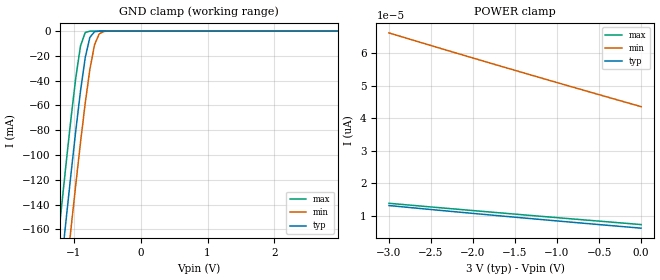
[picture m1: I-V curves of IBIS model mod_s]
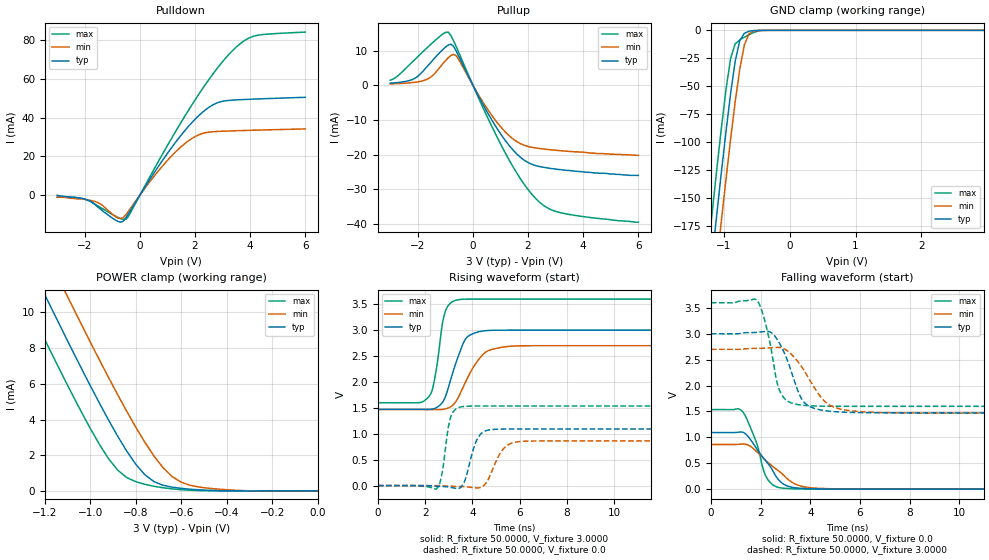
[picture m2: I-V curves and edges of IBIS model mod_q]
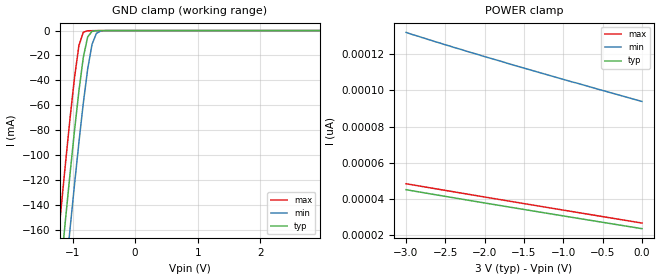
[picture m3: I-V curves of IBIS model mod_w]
| IBIS (I/O, Buffer, Information, Specification) Model, officially
| electronic behavioral standard for Buffer structures of digital pins.
[IBIS ver]  4.0
[File name] m95xxx_tssop8_3v.ibs
[File Rev]  16
[Date]  13 December 2012
[Source]   CAD & Design Services (Catania) - STMicroelectronics
[Notes]
   (Note1)  This IBIS model includes the TSSOP8 package parasitic data
   (Note2)  This IBIS model considers: VCC= 3.00(TYP), 2.70(MIN), 3.60(MAX)
   (Note3)  This IBIS model has some Notes about the non-monotonicity
   of the I-V curves, but they are not indicative of problems
   inside the model;
[Copyright] (c) 2012 STMicroelectronics
| - M95xxx EEPROM (F8H/P2 process)
| - Voltage Supply Range: 2.7V/3.6V
| - Package: TSSOP8
[Component] M95XXX
[Manufacturer] STMicroelectronics
[Package]
| variable   typ   min   max
R_pkg   0.0   0.0   0.0
L_pkg   0.0H   0.0H   0.0H
C_pkg   0.0F   0.0F   0.0F
[Pin]   signal_name   model_name   R_pin   L_pin   C_pin
1   SN   mod_s   NA   NA   NA
2   Q   mod_q   NA   NA   NA
3   WN   mod_w   NA   NA   NA
4   GND   GND   NA   NA   NA
5   D   mod_s   NA   NA   NA
6   C   mod_s   NA   NA   NA
7   HOLDN   mod_h   NA   NA   NA
8   VCC   POWER   NA   NA   NA
[Package Model]  182696_TSSOP8
[Define Package Model]  182696_TSSOP8
[Manufacturer]  STMicroelectronics
[OEM]  STMicroelectronics
[Description]  8 pin TSSOP package
[Number Of Pins]  8
[Pin Numbers]
|Pin Num   Terminal Name
1   | net1
2   | net2
3   | net3
4   | net4_GND
5   | net5
6   | net6
7   | net7
8   | net8_VDD
[Model Data]
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[End Model Data]
[End Package Model]
| Models and submodels in the file (4): mod_s (Input), mod_q (I/O), mod_w (Input), mod_h (Input)
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|   Model mod_s
[Model]   mod_s   | associated to PIN1 (S), PIN5 (D), PIN6 (CK)
Model_type Input
Vinl   =   0.90V
Vinh   =   2.10V
C_comp   2.120pF   2.024pF   2.323pF
[Temperature Range]  25.0000   85.0000   -40.0000
[Voltage Range]   3.0000V   2.7000V   3.6000V
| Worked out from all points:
|   GND clamp passes 1 mA (typ) near -0.70 V on its own axis
[GND_clamp]
|Voltage   I(typ)   I(min)   I(max)
-3V       -1.187A    -1.23A     -1.145A
-1.25V    -222.4mA   -267.4mA   -176.8mA
-1.18V    -185.7mA   -230.5mA   -140mA
-1.11V    -149.5mA   -194.1mA   -104.1mA
-1.04V    -114.1mA   -158.4mA   -69.45mA
-900mV    -48.41mA   -89.89mA   -11.98mA
-830mV    -21.59mA   -58.45mA   -1.177mA
-760mV    -5.046mA   -30.94mA   -53.02uA
-690mV    -552.5uA   -11.01mA   -2.192uA
-620mV    -47.07uA   -2.191mA   -90.25nA
-550mV    -3.895uA   -303.2uA   -3.716nA
2.95V     6.148pA    45.44pA    6.002pA
[POWER_clamp]
|Voltage   I(typ)   I(min)   I(max)
-3V       13.21pA    66.27pA    13.9pA
-2.32V    11.55pA    61pA       12.37pA
-1.56V    9.763pA    55.21pA    10.7pA
0V        6.257pA    43.6pA     7.361pA
|   Model mod_q
[Model]   mod_q
Model_type I/O
Polarity   Non-Inverting
Enable   Active-Low
Vinl   =   0.90V
Vinh   =   2.10V
Vmeas  =   1.50V
Cref   =   30pF
C_comp   2.925pF   2.667pF   3.207pF
[Temperature Range]  25.0000   85.0000   -40.0000
[Voltage Range]   3.0000V   2.7000V   3.6000V
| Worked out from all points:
|   slope of the pulldown table from 0 to 0.45 V, typ, clamps not added: 44.7 ohm
|   slope of the pullup table from 0 to 0.45 V, typ, clamps not added: 66.5 ohm
|   GND clamp passes 1 mA (typ) near -0.63 V on its own axis
|   POWER clamp passes 1 mA (typ) near -0.77 V on its own axis
|   rising waveform, R_fixture 50.0000, V_fixture 3.0000: 20-80 % time 660ps typ, 884ps min, 383ps max; typ from 1.47 V to 3 V
|   rising waveform, R_fixture 50.0000, V_fixture 0.0: 20-80 % time 417ps typ, 551ps min, 284ps max; typ from 0 V to 1.09 V
|   falling waveform, R_fixture 50.0000, V_fixture 0.0: 20-80 % time 951ps typ, 1.23ns min, 604ps max; typ from 1.09 V to 0 V
|   falling waveform, R_fixture 50.0000, V_fixture 3.0000: 20-80 % time 717ps typ, 1.03ns min, 501ps max; typ from 3 V to 1.47 V
[Pulldown]
|Voltage   I(typ)   I(min)   I(max)
-3V       0A         -1mA       -1mA
-2V       -2mA       -2.2mA     -2mA
-1.5V     -6.4mA     -4mA       -5.7mA
-800mV    -13.5mA    -11.76mA   -11.44mA
-500mV    -11.51mA   -9.918mA   -12.47mA
700mV     15.43mA    13mA       18.14mA
1.6V      32.77mA    26.26mA    40.04mA
2.5V      45.28mA    32.53mA    59.58mA
3.3V      48.97mA    33.16mA    73.69mA
3.8V      49.37mA    33.38mA    79.81mA
4.2V      49.6mA     33.54mA    82.29mA
6V        50.5mA     34.19mA    84.15mA
[Pullup]
|Voltage   I(typ)   I(min)   I(max)
-3V       607uA      390uA      1.431mA
-2.2V     1.638mA    771uA      6.685mA
-1.7V     5.035mA    1.591mA    10.53mA
-900mV    11.57mA    7.892mA    15.33mA
-800mV    11.85mA    8.576mA    14.37mA
-600mV    9.743mA    8.469mA    11.03mA
400mV     -6.056mA   -5.315mA   -7.07mA
1.2V      -16.2mA    -13.67mA   -19.91mA
1.8V      -21.26mA   -17.13mA   -27.87mA
2.3V      -23.22mA   -18.11mA   -32.85mA
3.2V      -24.36mA   -18.89mA   -36.79mA
6V        -26mA      -20.25mA   -39.5mA
[GND_clamp]
|Voltage   I(typ)   I(min)   I(max)
-3V       -1.27A     -1.311A    -1.233A
-1.25V    -242.6mA   -286.5mA   -202.2mA
-1.18V    -203.4mA   -247.3mA   -163mA
-1.11V    -164.8mA   -208.5mA   -124.5mA
-1.04V    -127mA     -170.4mA   -87.49mA
-900mV    -56.73mA   -97.48mA   -25.18mA
-830mV    -27.69mA   -63.94mA   -11.99mA
-760mV    -9.035mA   -34.5mA    -8.517mA
-690mV    -2.674mA   -12.96mA   -6.166mA
-620mV    -820uA     -3.056mA   -3.956mA
-480mV    -66.77uA   -203.2uA   -464.1uA
2.95V     219.9pA    2.348uA    145.8pA
[POWER_clamp]
|Voltage   I(typ)   I(min)   I(max)
-3V       59.85mA    62.21mA    57.45mA
-1.32V    14.15mA    16.63mA    11.63mA
-1.28V    13.09mA    15.58mA    10.57mA
-1.2V     10.99mA    13.48mA    8.479mA
-1.12V    8.922mA    11.4mA     6.427mA
-1.08V    7.9mA      10.37mA    5.424mA
-960mV    4.924mA    7.344mA    2.612mA
-880mV    3.078mA    5.401mA    1.172mA
-760mV    906.8uA    2.725mA    369.2uA
-640mV    211.2uA    805.3uA    114.6uA
-480mV    34.78uA    150.4uA    8.134uA
0V        232.7pA    560.7pA    273.1pA
[Ramp]
| variable   typ   min   max
dV/dt_r  0.6562/0.4689n   0.5173/0.6028n   0.9211/0.3567n
dV/dt_f  0.9143/0.7906n   0.7365/1.0864n   1.2006/0.5636n
R_load = 50.0000
[Rising Waveform]
R_fixture= 50.0000
V_fixture= 3.0000
V_fixture_min= 2.7000
V_fixture_max= 3.6000
|time   V(typ)   V(min)   V(max)
0s        1.473V     1.468V     1.599V
1.815ns   1.472V     1.468V     1.604V
2.175ns   1.471V     1.467V     1.726V
2.415ns   1.491V     1.466V     2.081V
2.805ns   1.659V     1.475V     3.282V
3.285ns   2.342V     1.61V      3.575V
3.795ns   2.872V     2.078V     3.599V
4.455ns   2.985V     2.534V     3.6V
5.055ns   2.999V     2.652V     3.6V
15ns      3V         2.7V       3.6V
[Rising Waveform]
R_fixture= 50.0000
V_fixture= 0.0
V_fixture_min= 0.0
V_fixture_max= 0.0
|time   V(typ)   V(min)   V(max)
0s        8.564nV    55.05nV    9.295nV
2.46ns    -11.03mV   -184.3uV   -68.49mV
2.685ns   -15.37mV   -2.735mV   159.4mV
3.075ns   -33.1mV    -10.87mV   1.31V
3.495ns   -38.76mV   -16.85mV   1.517V
4.185ns   876.7mV    -44.76mV   1.536V
4.665ns   1.071V     111.9mV    1.536V
5.325ns   1.092V     716mV      1.536V
5.955ns   1.093V     848.2mV    1.536V
15ns      1.093V     862.3mV    1.536V
[Falling Waveform]
R_fixture= 50.0000
V_fixture= 0.0
V_fixture_min= 0.0
V_fixture_max= 0.0
|time   V(typ)   V(min)   V(max)
0s        1.093V     862.3mV    1.536V
1.08ns    1.098V     864.3mV    1.553V
1.275ns   1.1V       870.7mV    1.496V
1.815ns   801.6mV    738mV      926.3mV
2.205ns   547.8mV    556.1mV    259.5mV
2.445ns   394.9mV    455.4mV    102.2mV
2.745ns   170.7mV    345.5mV    30.78mV
3.405ns   25.81mV    97.17mV    6.031mV
4.23ns    6.556mV    18.46mV    816.1uV
15ns      4.641nV    50.56nV    7.037nV
[Falling Waveform]
R_fixture= 50.0000
V_fixture= 3.0000
V_fixture_min= 2.7000
V_fixture_max= 3.6000
|time   V(typ)   V(min)   V(max)
0s        3V         2.7V       3.6V
1.89ns    3.029V     2.718V     3.624V
2.265ns   3.048V     2.724V     3.068V
2.73ns    2.844V     2.736V     1.95V
3.3ns     2.178V     2.574V     1.655V
3.6ns     1.787V     2.399V     1.626V
3.9ns     1.618V     2.171V     1.613V
4.59ns    1.516V     1.689V     1.602V
5.34ns    1.486V     1.534V     1.6V
15ns      1.473V     1.468V     1.599V
|   Model mod_w
[Model]   mod_w
Model_type Input
Vinl   =   0.90V
Vinh   =   2.10V
C_comp   2.120pF   2.024pF   2.323pF
[Temperature Range]  25.0000   85.0000   -40.0000
[Voltage Range]   3.0000V   2.7000V   3.6000V
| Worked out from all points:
|   GND clamp passes 1 mA (typ) near -0.70 V on its own axis
[GND_clamp]
|Voltage   I(typ)   I(min)   I(max)
-3V       -1.188A    -1.23A     -1.146A
-1.25V    -222.7mA   -267.6mA   -177.1mA
-1.18V    -185.9mA   -230.7mA   -140.3mA
-1.11V    -149.6mA   -194.3mA   -104.3mA
-1.04V    -114.2mA   -158.5mA   -69.64mA
-900mV    -48.52mA   -89.98mA   -12.13mA
-830mV    -21.68mA   -58.53mA   -1.302mA
-760mV    -5.115mA   -31mA      -157.1uA
-690mV    -601.3uA   -11.05mA   -84.87uA
-620mV    -77.84uA   -2.215mA   -61.81uA
-550mV    -19.41uA   -316.9uA   -41.57uA
2.95V     23.17pA    96.93pA    21.99pA
[POWER_clamp]
|Voltage   I(typ)   I(min)   I(max)
-3V       45.07pA    132.1pA    48.38pA
-2.4V     40.65pA    123.9pA    43.95pA
-1.72V    35.72pA    115.1pA    38.99pA
-880mV    29.72pA    104.6pA    32.92pA
0V        23.52pA    93.89pA    26.62pA
